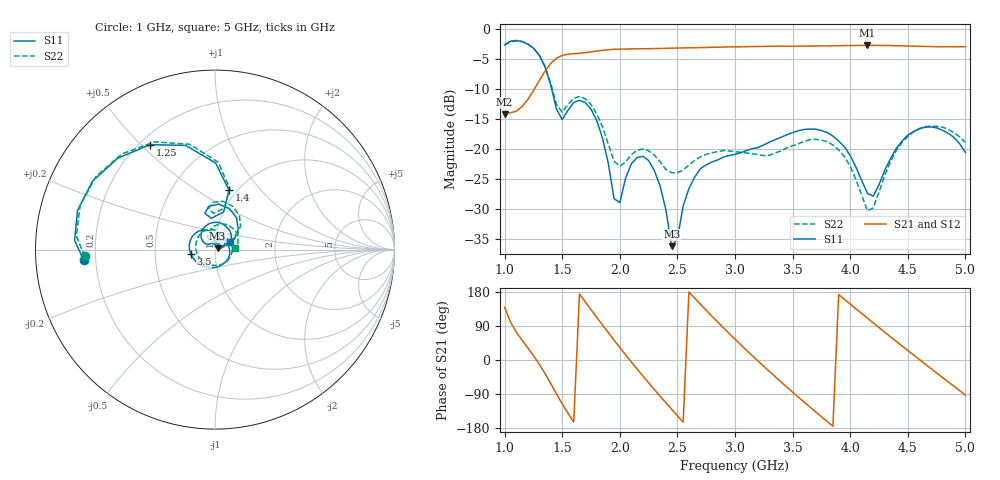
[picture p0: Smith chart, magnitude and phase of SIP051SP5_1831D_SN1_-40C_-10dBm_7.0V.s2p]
# GHz  S  dB  R  50
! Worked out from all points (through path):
!   81 points, 1 GHz to 5 GHz, reference 50 ohm
!   highest |S21| = -2.79 dB at 4.15 GHz (marker M1); lowest = -14.2 dB at 1 GHz (marker M2)
!   lowest |S11| = -36.1 dB at 2.45 GHz (marker M3), VSWR 1.03, Z = 51.4 + j0.709 ohm
!   |S11| at or under -10 dB: 1.408 GHz to end of sweep
!   |S22| runs from -30.3 to -2.0 dB; largest |S21 - S12| = 0.0027
!   S11 on the Smith chart (normalised r, x): 1 GHz: 0.15, -0.04; 1.25 GHz: 0.24, +0.53; 1.4 GHz: 0.92, +0.69; 3.5 GHz: 0.76, -0.04; 5 GHz: 1.18, +0.10
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1  -2.69 -175.3  -14.21 139.1  -14.18 139.2  -2.77 -177.0
1.25  -3.25 121.7  -10.31 11.7  -10.33 11.6  -3.24 119.3
1.4  -9.36 76.8  -5.80 -61.8  -5.80 -61.8  -9.10 76.4
1.5  -15.11 96.7  -4.46 -115.6  -4.45 -115.6  -13.87 92.8
1.7  -12.29 71.1  -4.00 153.5  -4.00 153.5  -11.66 67.5
1.85  -18.19 28.3  -3.62 92.3  -3.62 92.2  -16.32 33.8
1.95  -28.24 30.7  -3.45 52.4  -3.46 52.4  -22.02 37.3
2.05  -24.86 94.4  -3.40 13.7  -3.40 13.8  -22.13 62.7
2.2  -21.21 58.5  -3.36 -42.0  -3.36 -42.0  -20.01 50.4
2.35  -26.12 18.2  -3.31 -95.5  -3.29 -95.5  -22.10 34.6
2.45  -36.12 26.2  -3.26 -130.1  -3.26 -130.1  -23.93 38.5
2.65  -24.65 68.4  -3.18 163.2  -3.18 163.2  -21.89 43.2
2.85  -21.80 -0.0  -3.11 100.1  -3.10 100.1  -20.42 14.2
3  -20.88 -49.3  -3.04 54.9  -3.04 55.0  -20.44 -16.9
3.25  -19.31 -117.2  -2.96 -16.9  -2.96 -16.9  -21.09 -91.8
3.5  -17.27 -168.9  -2.94 -84.8  -2.93 -84.9  -19.45 -179.5
3.7  -16.71 150.1  -2.91 -136.8  -2.90 -136.9  -18.39 123.8
3.9  -18.67 111.7  -2.85 172.6  -2.85 172.6  -20.12 78.1
4.15  -27.37 107.3  -2.79 110.3  -2.78 110.3  -30.27 74.2
4.35  -21.58 145.7  -2.82 61.2  -2.84 61.3  -22.08 118.3
4.65  -16.38 93.7  -2.97 -10.4  -2.98 -10.5  -16.30 66.4
5  -20.55 25.8  -3.02 -92.8  -3.02 -92.8  -18.89 3.2
